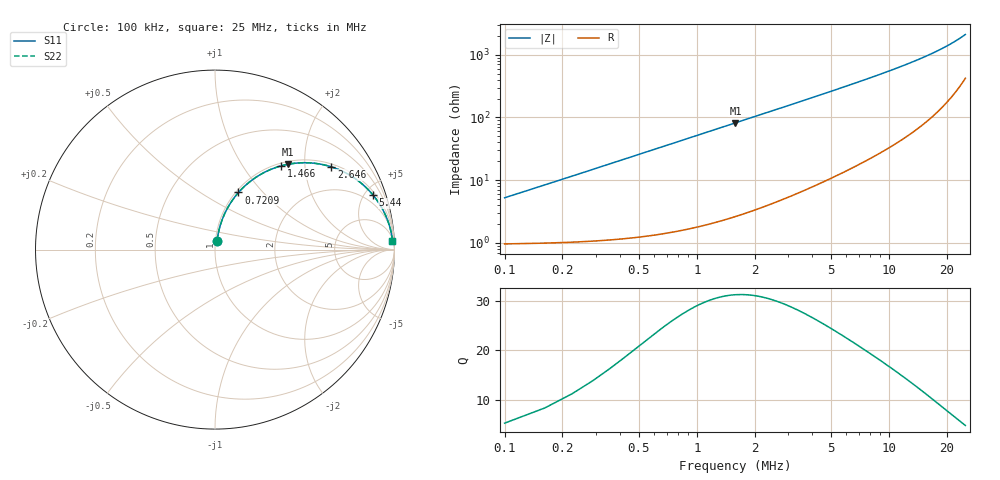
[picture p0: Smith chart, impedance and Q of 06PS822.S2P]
! Coilcraft 0603PS-822 Power Chip Inductor
! 19 February 2003
# MHZ S MA R 50
!Freq  MagS11  AngS11  MagS21  AngS21  MagS12  AngS12  MagS22  AngS22
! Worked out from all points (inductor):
!   403 points, 100 kHz to 25 MHz, reference 50 ohm
!   read as one part in series: L = 8.2 uH near 224.2 kHz
!   highest Q = 31.2 at 1.59 MHz (marker M1), where L = 8.21 uH
!   S11 on the Smith chart (normalised r, x): 100 kHz: 1.02, +0.10; 720.9 kHz: 1.03, +0.74; 1.466 MHz: 1.05, +1.51; 2.646 MHz: 1.09, +2.74; 5.44 MHz: 1.24, +5.71; 25 MHz: 9, +41
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0.1  0.05185 76.5  0.9892 -2.9  0.9892 -2.9  0.05185 76.5
0.16209  0.08299 78.5  0.9868 -4.7  0.9868 -4.7  0.08299 78.5
0.28627  0.1448 77.6  0.9791 -8.3  0.9791 -8.3  0.1448 77.6
0.34836  0.1751 76.4  0.9738 -10.1  0.9738 -10.1  0.1751 76.4
0.41045  0.2049 75.1  0.9676 -11.8  0.9676 -11.8  0.2049 75.1
0.53463  0.2628 72.1  0.9529 -15.2  0.9529 -15.2  0.2628 72.1
0.7209  0.3441 67.6  0.9256 -20.1  0.9256 -20.1  0.3441 67.6
0.84508  0.3943 64.7  0.9047 -23.2  0.9047 -23.2  0.3943 64.7
1.03135  0.4631 60.5  0.8706 -27.6  0.8706 -27.6  0.4631 60.5
1.46598  0.5942 51.7  0.7854 -36.4  0.7854 -36.4  0.5942 51.7
1.59016  0.6247 49.5  0.7611 -38.6  0.7611 -38.6  0.6247 49.5
2.08688  0.7216 42.0  0.6693 -46.2  0.6693 -46.2  0.7216 42.0
2.64569  0.7949 35.5  0.5806 -52.6  0.5806 -52.6  0.7949 35.5
3.39077  0.8564 29.1  0.4867 -58.9  0.4867 -58.9  0.8564 29.1
4.26003  0.8989 23.9  0.4049 -63.9  0.4049 -63.9  0.8989 23.9
5.43974  0.9315 19.0  0.3262 -68.5  0.3262 -68.5  0.9315 19.0
6.74363  0.9515 15.4  0.266 -71.9  0.266 -71.9  0.9515 15.4
8.42006  0.9659 12.3  0.2127 -74.7  0.2127 -74.7  0.9659 12.3
12.58009  0.981 7.8  0.1362 -78.1  0.1362 -78.1  0.981 7.8
16.74012  0.9865 5.4  0.09411 -79.1  0.09411 -79.1  0.9865 5.4
20.90015  0.9887 3.8  0.0666 -78.4  0.0666 -78.4  0.9887 3.8
25  0.9895 2.6  0.04694 -75.8  0.04694 -75.8  0.9895 2.6
